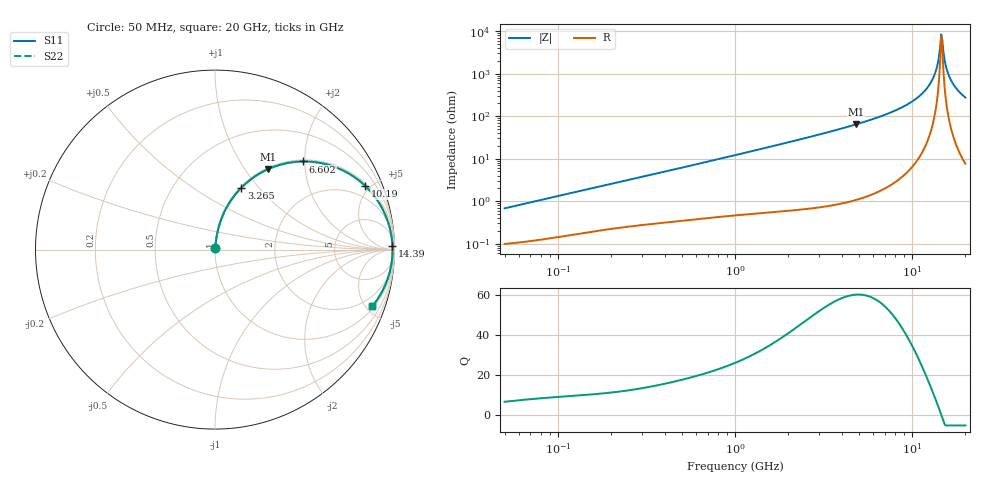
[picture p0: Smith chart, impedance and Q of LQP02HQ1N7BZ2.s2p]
!Murata Part Number: LQP02HQ1N7BZ2
!These Parameters are Measured in Series Mode Connection
!  o--[Z]--o
!Port1  Port2
!  o-------o
!Freq. Start=50[MHz] Stop=20[GHz], 401[Steps]
# Hz S RI R 50
!Freq.(Hz) S11(Real) S11(Imag) S21(Real) S21(Imag) S12(Real) S12(Imag) S22(Real) S22(Imag)
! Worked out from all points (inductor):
!   401 points, 50 MHz to 20 GHz, reference 50 ohm
!   read as one part in series: L = 2.12 nH near 51.52 MHz
!   highest Q = 60.2 at 4.82 GHz (marker M1), where L = 2.11 nH
!   self-resonance near 14.6 GHz
!   S11 on the Smith chart (normalised r, x): 50 MHz: 1.00, +0.01; 3.265 GHz: 1.02, +0.82; 6.602 GHz: 1.03, +1.96; 10.19 GHz: 1.14, +4.67; 14.39 GHz: 37, +73; 20 GHz: 1.15, -5.50
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5e7  0.00103 0.00667  0.999 -0.00667  0.999 -0.00667  0.00103 0.00667
1.364002e8  0.00205 0.0176  0.9979 -0.0176  0.9979 -0.0176  0.00205 0.0176
3.721004e8  0.00509 0.0455  0.9949 -0.0455  0.9949 -0.0455  0.00509 0.0455
1e9  0.0187 0.1178  0.9813 -0.1178  0.9813 -0.1178  0.0187 0.1178
2.728004e9  0.106 0.2979  0.894 -0.2979  0.894 -0.2979  0.106 0.2979
3.265178e9  0.147 0.3451  0.853 -0.3451  0.853 -0.3451  0.147 0.3451
4.81993e9  0.294 0.4474  0.706 -0.4474  0.706 -0.4474  0.294 0.4474
6.601595e9  0.4905 0.4911  0.5095 -0.4911  0.5095 -0.4911  0.4905 0.4911
7.442007e9  0.5834 0.4835  0.4166 -0.4835  0.4166 -0.4835  0.5834 0.4835
1.019291e10  0.8377 0.354  0.1623 -0.354  0.1623 -0.354  0.8377 0.354
1.166392e10  0.9244 0.2429  0.0756 -0.2429  0.0756 -0.2429  0.9244 0.2429
1.295331e10  0.9693 0.1372  0.0307 -0.1372  0.0307 -0.1372  0.9693 0.1372
1.375312e10  0.9838 0.0719  0.0162 -0.0719  0.0162 -0.0719  0.9838 0.0719
1.438523e10  0.9887 0.0216  0.0113 -0.0216  0.0113 -0.0216  0.9887 0.0216
1.460232e10  0.9892 0.00475  0.0108 -0.00475  0.0108 -0.00475  0.9892 0.00475
1.482269e10  0.9891 -0.0121  0.0109 0.0121  0.0109 0.0121  0.9891 -0.0121
1.504638e10  0.9885 -0.029  0.0115 0.029  0.0115 0.029  0.9885 -0.029
1.550395e10  0.9855 -0.0626  0.0145 0.0626  0.0145 0.0626  0.9855 -0.0626
1.573793e10  0.9831 -0.0792  0.0169 0.0792  0.0169 0.0792  0.9831 -0.0792
1.670968e10  0.9681 -0.1445  0.0319 0.1445  0.0319 0.1445  0.9681 -0.1445
1.828096e10  0.9302 -0.2357  0.0698 0.2357  0.0698 0.2357  0.9302 -0.2357
2e10  0.8767 -0.3152  0.1233 0.3152  0.1233 0.3152  0.8767 -0.3152
